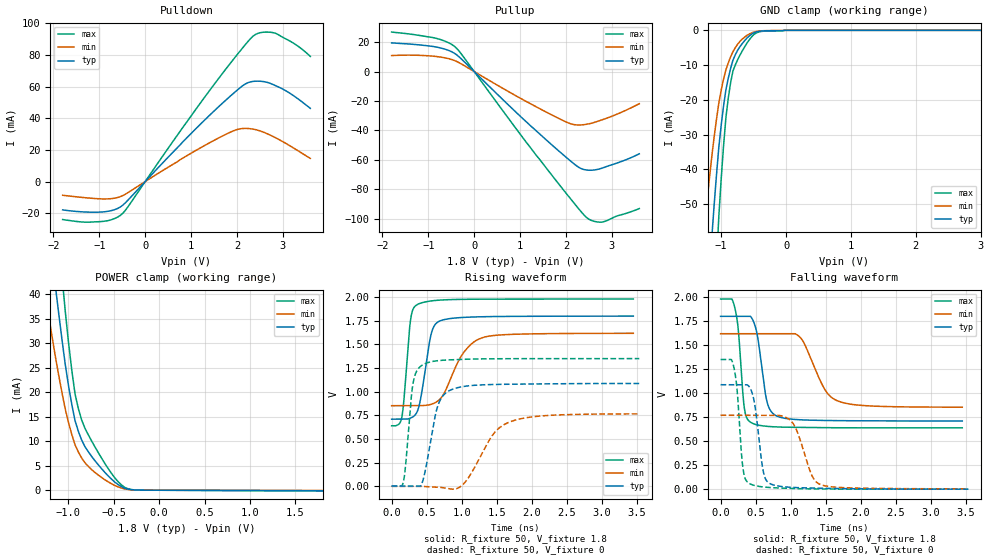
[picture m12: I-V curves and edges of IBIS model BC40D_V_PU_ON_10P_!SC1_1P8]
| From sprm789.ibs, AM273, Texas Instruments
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|   Model Cell BC40D_V_PU_ON_10P_!SC1_1P8
|BC40D_V_PU_ON_10P_!SC1_1P8
[Model]   BC40D_V_PU_ON_10P_!SC1_1P8
Model_type   I/O
Polarity   Non-Inverting
Enable   Active-Low
Vinl =  0.63
Vinh =  1.17
Cref =  15pF
Rref =  100.0000M
Vref =  0V
Vmeas =  0.9
C_comp   2.290246p   2.205796p   2.292736p
|[Input load] weak_pu_on
|[Output drive] fast
|[supplytol] 10
|[temp] ind
[Model Spec]
Vinl   0.63   0.567   0.693
Vinh   1.17   1.053   1.287
[Temperature Range]   25   125   -40
[Voltage Range]   1.8   1.62   1.98
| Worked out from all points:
|   slope of the pulldown table from 0 to 0.27 V, typ, clamps not added: 32.2 ohm
|   slope of the pullup table from 0 to 0.27 V, typ, clamps not added: 32.5 ohm
|   GND clamp passes 1 mA (typ) near -0.52 V on its own axis
|   POWER clamp passes 1 mA (typ) near -0.44 V on its own axis
|   rising waveform, R_fixture 50, V_fixture 1.8: 20-80 % time 141ps typ, 321ps min, 87.2ps max; typ from 0.71 V to 1.8 V
|   rising waveform, R_fixture 50, V_fixture 0: 20-80 % time 174ps typ, 380ps min, 98.7ps max; typ from 0.003 V to 1.09 V
|   falling waveform, R_fixture 50, V_fixture 1.8: 20-80 % time 128ps typ, 290ps min, 84ps max; typ from 1.8 V to 0.711 V
|   falling waveform, R_fixture 50, V_fixture 0: 20-80 % time 111ps typ, 211ps min, 81ps max; typ from 1.09 V to 0.002 V
| Nom Voltages:
|   VDD=1.1001, VDDS=1.8, VDDS18=1.8, ESD_BIASFET=0, VSS=0, VSSS=0
| Min Voltages:
|   VDD=0.99, VDDS=1.62, VDDS18=1.62, ESD_BIASFET=0, VSS=0, VSSS=0
| Max Voltages:
|   VDD=1.21, VDDS=1.98, VDDS18=1.98, ESD_BIASFET=0, VSS=0, VSSS=0
[POWER_clamp]
|   voltage   I(typ)   I(min)   I(max)
-1.8V     158.8mA    112.5mA    219.8mA
-1.255V   59.97mA    40.01mA    84.9mA
-1.145V   41.92mA    27.42mA    59.75mA
-1.109V   36.32mA    23.63mA    51.82mA
-1.073V   30.96mA    20.05mA    44.15mA
-1.036V   25.83mA    16.67mA    36.75mA
-963.6mV  17.54mA    11.39mA    24.55mA
-890.9mV  12.01mA    7.801mA    16.66mA
-818.2mV  8.875mA    5.6mA      12.63mA
-563.6mV  2.954mA    1.727mA    4.458mA
-272.7mV  55.97uA    39.41uA    57.82uA
1.8V      -99.94uA   -59.68uA   -146.8uA
[Pulldown]
|   voltage   I(typ)   I(min)   I(max)
-1.8V     -17.92mA   -8.674mA   -24.03mA
-927.3mV  -19.22mA   -10.99mA   -25.21mA
-654.5mV  -17.65mA   -10.46mA   -23.22mA
-490.9mV  -14.97mA   -8.904mA   -20.12mA
818.2mV   25.06mA    14.78mA    34.16mA
1.691V    49.7mA     28.87mA    68.59mA
2.127V    60.63mA    33.53mA    84.59mA
2.4V      63.43mA    32.84mA    92.9mA
2.618V    62.99mA    30.74mA    94.47mA
2.836V    60.69mA    27.76mA    93.76mA
3.273V    53.49mA    20.53mA    86.73mA
3.6V      46.26mA    14.64mA    79.11mA
[Pullup]
|   voltage   I(typ)   I(min)   I(max)
-1.8V     19.47mA    10.86mA    26.81mA
-818.2mV  16.61mA    10.18mA    22.5mA
-545.5mV  14.21mA    8.665mA    19.39mA
-381.8mV  11.35mA    6.855mA    15.77mA
1.036V    -31.31mA   -18.66mA   -43.94mA
1.909V    -55.72mA   -32.86mA   -78.99mA
2.182V    -62.87mA   -36.1mA    -89.59mA
2.345V    -66.12mA   -36.26mA   -95.76mA
2.455V    -66.95mA   -35.82mA   -99.33mA
2.618V    -66.9mA    -34.58mA   -101.8mA
2.782V    -65.73mA   -32.89mA   -102.4mA
3.6V      -55.92mA   -21.86mA   -93.15mA
[GND_clamp]
|   voltage   I(typ)   I(min)   I(max)
-1.8V     -270.2mA   -170.2mA   -430.1mA
-1.255V   -91.68mA   -55.92mA   -148.5mA
-1.145V   -59.94mA   -36.46mA   -97.15mA
-1.109V   -50.51mA   -30.84mA   -81.62mA
-1.073V   -41.77mA   -25.67mA   -67.14mA
-1.036V   -33.71mA   -20.94mA   -53.69mA
-927.3mV  -17.15mA   -11.38mA   -25.2mA
-854.5mV  -10.96mA   -7.657mA   -15.09mA
-781.8mV  -7.031mA   -4.995mA   -9.958mA
-563.6mV  -1.569mA   -1.036mA   -2.651mA
-18.18mV  0A         0A         0A
3.6V      0A         0A         0A
[Ramp]
| variable   typ   min   max
dV/dt_f  0.6650793/0.13041675n 0.47054236/0.29704481n 0.81398134/85.756989p
dV/dt_r 0.66369803/0.17655946n 0.48061665/0.39565974n 0.81803201/99.446129p
R_load = 50
[Rising Waveform]
R_fixture = 50
V_fixture = 1.8
V_fixture_min = 1.62
V_fixture_max = 1.98
|   time   V(typ)   V(min)   V(max)
0s        710.4mV    852.8mV    640.4mV
144.3ps   710.4mV    852.8mV    725.7mV
175.6ps   710.4mV    852.8mV    911.9mV
270.1ps   722mV      852.8mV    1.757V
370ps     797.4mV    852.8mV    1.923V
562.2ps   1.602V     867mV      1.96V
684.5ps   1.747V     917.1mV    1.969V
1.012ns   1.785V     1.397V     1.977V
1.288ns   1.793V     1.569V     1.979V
3.453ns   1.8V       1.618V     1.98V
[Rising Waveform]
R_fixture = 50
V_fixture = 0
V_fixture_min = 0
V_fixture_max = 0
|   time   V(typ)   V(min)   V(max)
0s        2.784mV    0V         2.119mV
166.4ps   2.784mV    0V         43.04mV
306.9ps   2.784mV    0V         1.091V
461ps     100.5mV    0V         1.292V
655.4ps   840.3mV    -8.842mV   1.328V
846.9ps   1.02V      -28.35mV   1.338V
1.045ns   1.058V     39.43mV    1.344V
1.45ns    1.077V     549.2mV    1.349V
1.678ns   1.08V      678mV      1.35V
3.539ns   1.088V     766.3mV    1.351V
[Falling Waveform]
R_fixture = 50
V_fixture = 1.8
V_fixture_min = 1.62
V_fixture_max = 1.98
|   time   V(typ)   V(min)   V(max)
0s        1.8V       1.619V     1.979V
200.7ps   1.8V       1.619V     1.897V
252.9ps   1.8V       1.619V     1.661V
340.6ps   1.8V       1.619V     841.1mV
445.7ps   1.782V     1.619V     691.1mV
662.6ps   914.6mV    1.619V     655.8mV
801.7ps   763.7mV    1.619V     649.7mV
1.144ns   723.8mV    1.575V     644.9mV
1.675ns   715.2mV    919.9mV    641.1mV
3.453ns   711.4mV    854.9mV    639.8mV
[Falling Waveform]
R_fixture = 50
V_fixture = 0
V_fixture_min = 0
V_fixture_max = 0
|   time   V(typ)   V(min)   V(max)
0s        1.089V     771mV      1.351V
188.4ps   1.089V     771mV      1.276V
237.3ps   1.089V     771mV      1.026V
319ps     1.089V     771mV      224.9mV
421.8ps   1.054V     771mV      57.69mV
608.8ps   191.6mV    771mV      25.46mV
717.5ps   56.12mV    771mV      18.73mV
1.033ns   20.81mV    688.6mV    9.86mV
1.431ns   11.84mV    49.28mV    4.351mV
3.539ns   2.48mV     4.818mV    2.572mV
